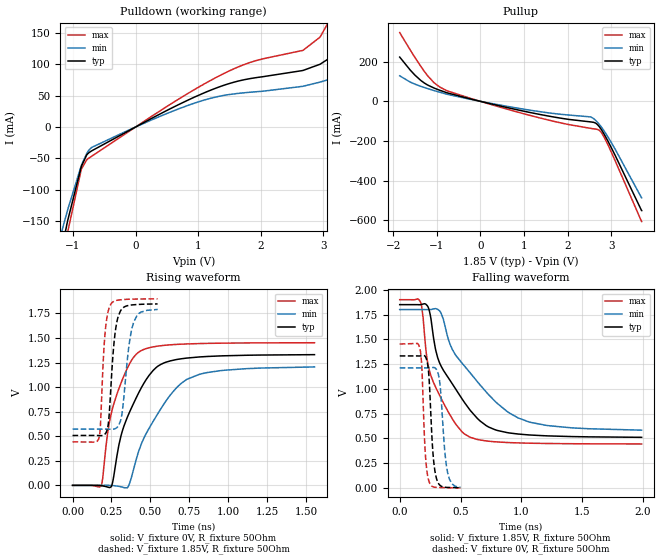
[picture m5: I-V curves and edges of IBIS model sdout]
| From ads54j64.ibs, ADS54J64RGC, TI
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|   sdout Model
[Model]   sdout
Model_type   Output
Polarity   Non-Inverting
Vmeas = 0.925
Vref = 0
Cref = 2pF
Rref = 50
|   typ   min   max
|   (nom PVT)   (fast PVT)   (slow PVT)
C_comp   4.012e-13   3.389e-13   4.824e-13
| Where nom  PVT is Nominal Process, 1.85V, 27C
|   Fast PVT is Strong Process,  1.9V, -40C
|   Slow PVT is Weak Process,   1.8V, 125C
[Voltage Range]   1.85   1.8   1.9
|Junction Temperature
[Temperature Range]   27   125   -40
[Pullup Reference]   1.85   1.8   1.9
[Pulldown Reference]   0   0   0
[Power Clamp Reference]   1.85   1.8   1.9
[GND Clamp Reference]   0   0   0
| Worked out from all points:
|   slope of the pulldown table from 0 to 0.278 V, typ, clamps not added: 18.6 ohm
|   slope of the pullup table from 0 to 0.278 V, typ, clamps not added: 19.2 ohm
|   falling waveform, V_fixture 1.85V, R_fixture 50Ohm: 20-80 % time 312ps typ, 441ps min, 214ps max; typ from 1.85 V to 0.511 V
|   rising waveform, V_fixture 0V, R_fixture 50Ohm: 20-80 % time 186ps typ, 247ps min, 135ps max; typ from 0 V to 1.33 V
|   rising waveform, V_fixture 1.85V, R_fixture 50Ohm: 20-80 % time 38.1ps typ, 50.6ps min, 29.6ps max; typ from 0.508 V to 1.85 V
|   falling waveform, V_fixture 0V, R_fixture 50Ohm: 20-80 % time 36.2ps typ, 44.5ps min, 29.9ps max; typ from 1.33 V to 0.002 V
[Pulldown]
|   Voltage   I(typ)   I(min)   I(max)
-1.85V    -496.2mA   -443.4mA   -547.4mA
-1.481V   -340.1mA   -276.7mA   -381.5mA
-1.084V   -149.2mA   -131.8mA   -167.3mA
-862.1mV  -61.8mA    -60.3mA    -66.32mA
-778.4mV  -44.09mA   -41.72mA   -51.99mA
-703.4mV  -38.09mA   -32.62mA   -46.73mA
1.091V    54.45mA    42.97mA    68.58mA
1.813V    77.09mA    55.46mA    102.6mA
2.677V    90.52mA    65.23mA    122.7mA
3.099V    110.3mA    76.41mA    170.9mA
3.471V    166.5mA    102.1mA    268.1mA
3.7V      221.6mA    135.9mA    337.4mA
[Pullup]
|   Voltage   I(typ)   I(min)   I(max)
-1.85V    223.4mA    128.9mA    347.2mA
-1.504V   133mA      86.98mA    222.7mA
-1.198V   81.03mA    63.47mA    126.3mA
-1.058V   66.59mA    53.96mA    93.01mA
-791.8mV  45.14mA    37.31mA    56.23mA
1.147V    -56.77mA   -45.04mA   -71.74mA
2.535V    -104.2mA   -78.94mA   -136.8mA
2.641V    -109.8mA   -95.38mA   -140.2mA
2.729V    -128.4mA   -116.8mA   -146.5mA
2.864V    -175.3mA   -157.8mA   -191.5mA
3.098V    -275.8mA   -244.4mA   -303.1mA
3.7V      -552mA     -487.7mA   -607.3mA
[Ramp]
R_load = 50
|   typ   min   max
dV/dt_r   0.799474/1.8695e-10   0.727094/2.4876e-10   0.871468/1.35258e-10
dV/dt_f   0.805352/3.13752e-10   0.736463/4.47134e-10   0.874231/2.1456e-10
[Falling Waveform]
V_fixture = 1.85V
V_fixture_min = 1.8V
V_fixture_max = 1.9V
R_fixture = 50Ohm
|   Time   V(typ)   V(min)   V(max)
0s        1.85V      1.8V       1.9V
170.3ps   1.85V      1.8V       1.876V
192.5ps   1.856V     1.8V       1.717V
229.1ps   1.835V     1.799V     1.27V
326.2ps   1.267V     1.789V     938.8mV
432.4ps   1.05V      1.398V     697.5mV
571.6ps   795.9mV    1.173V     515.9mV
731.6ps   614.5mV    940.4mV    471.7mV
1.057ns   535.5mV    668.7mV    451.9mV
1.988ns   511mV      583.1mV    443.8mV
[Rising Waveform]
V_fixture = 0V
V_fixture_min = 0V
V_fixture_max = 0V
R_fixture = 50Ohm
|   Time   V(typ)   V(min)   V(max)
0s        86.46nV    542.2nV    588.8nV
183.9ps   -3.181mV   -30.63uV   -4.238mV
225.4ps   -17.4mV    442.3uV    532.3mV
264.9ps   93.78mV    -3.226mV   827.7mV
312ps     508.5mV    -14.47mV   1.044V
357.4ps   713.4mV    -12.69mV   1.21V
443.3ps   997.4mV    426.8mV    1.373V
549.3ps   1.214V     733.5mV    1.418V
733.8ps   1.296V     1.079V     1.44V
1.555ns   1.331V     1.206V     1.452V
[Rising Waveform]
V_fixture = 1.85V
V_fixture_min = 1.8V
V_fixture_max = 1.9V
R_fixture = 50Ohm
|   Time   V(typ)   V(min)   V(max)
0s        507.7mV    572.5mV    442.9mV
168.8ps   507mV      572.5mV    476.5mV
179.5ps   506.1mV    572.5mV    620.2mV
208.2ps   521.7mV    572.8mV    1.535V
229.9ps   627.9mV    572.2mV    1.778V
245.4ps   974.1mV    571.2mV    1.843V
272.3ps   1.537V     576.5mV    1.878V
306.9ps   1.773V     650.1mV    1.889V
391.9ps   1.838V     1.656V     1.896V
546.6ps   1.847V     1.791V     1.899V
[Falling Waveform]
V_fixture = 0V
V_fixture_min = 0V
V_fixture_max = 0V
R_fixture = 50Ohm
|   Time   V(typ)   V(min)   V(max)
0s        1.332V     1.212V     1.452V
166.1ps   1.332V     1.212V     1.406V
182.1ps   1.335V     1.212V     1.211V
221.6ps   1.293V     1.211V     190mV
240.9ps   1.115V     1.212V     64.78mV
273.5ps   348.7mV    1.216V     11.96mV
304.7ps   85.17mV    1.19V      5.239mV
333.1ps   24.3mV     1.023V     4.314mV
391.9ps   5.059mV    166mV      2.489mV
499.4ps   2.325mV    6.087mV    1.029mV
